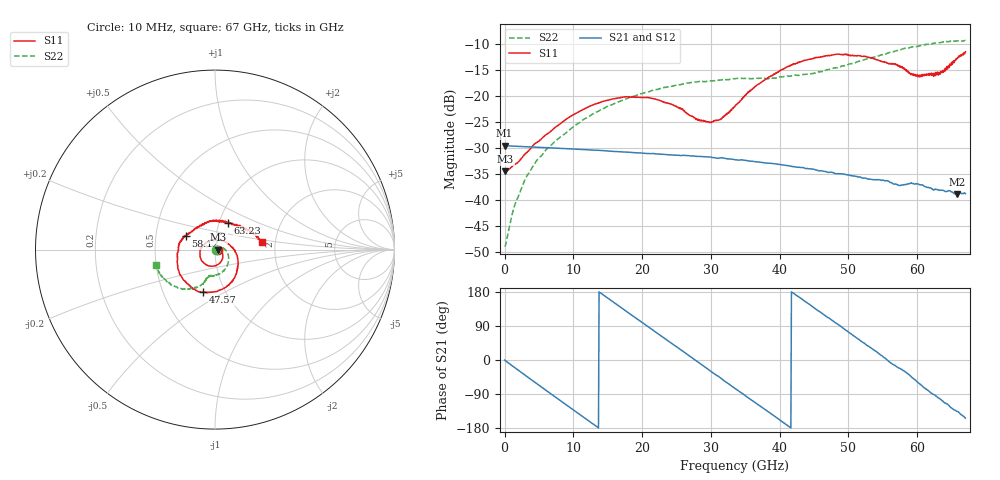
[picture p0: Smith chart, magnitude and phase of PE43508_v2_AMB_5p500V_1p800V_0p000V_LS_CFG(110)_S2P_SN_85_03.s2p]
!Keysight Technologies,N5227A,US51270237,A.10.43.00
!Date: Wednesday, August 22, 2018 17:18:10
!Correction: S11(Full 2 Port(1,3))
!S31(Full 2 Port(1,3))
!S13(Full 2 Port(1,3))
!S33(Full 2 Port(1,3))
!S2P File: Measurements: S11, S31, S13, S33:
# Hz S  dB  R 50
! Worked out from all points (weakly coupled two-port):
!   801 points, 10 MHz to 67 GHz, reference 50 ohm
!   highest |S21| = -29.57 dB at 10 MHz (marker M1); lowest = -38.9 dB at 65.83 GHz (marker M2)
!   lowest |S11| = -34.5 dB at 93.74 MHz (marker M3), VSWR 1.04, Z = 51.9 + j0.00866 ohm
!   |S11| at or under -10 dB: start of sweep to end of sweep
!   |S22| runs from -48.9 to -9.3 dB; largest |S21 - S12| = 0.0002
!   S11 on the Smith chart (normalised r, x): 10 MHz: 1.04, -0.00; 47.57 GHz: 0.79, -0.40; 58.12 GHz: 0.71, +0.11; 63.23 GHz: 1.10, +0.34; 67 GHz: 1.70, +0.15
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1e7  -34.43 -1.1  -29.57 -0.2  -29.58 -0.2  -48.82 -2.1
9.37375e7  -34.50 0.3  -29.59 -1.4  -29.60 -1.4  -48.90 7.8
1.68475e9  -33.03 3.3  -29.70 -22.8  -29.70 -22.9  -40.24 46.7
3.02455e9  -31.17 -0.3  -29.78 -40.6  -29.78 -40.6  -35.96 43.8
4.36435e9  -29.25 -7.2  -29.86 -58.2  -29.86 -58.2  -33.03 37.6
7.295162e9  -26.14 -28.8  -30.05 -96.6  -30.05 -96.5  -28.81 23.4
1.123082e10  -22.73 -61.1  -30.31 -147.7  -30.32 -147.7  -24.82 -1.0
1.74274e10  -20.22 -111.6  -30.78 132.2  -30.78 132.2  -20.68 -34.1
2.236791e10  -20.78 -154.8  -31.20 68.5  -31.19 68.5  -18.70 -57.0
2.973681e10  -25.07 96.9  -31.76 -26.3  -31.76 -26.3  -17.10 -82.8
3.132782e10  -24.56 63.7  -31.93 -46.3  -31.94 -46.3  -16.94 -87.6
3.3505e10  -22.04 24.3  -32.27 -75.1  -32.28 -75.2  -16.69 -93.3
3.836178e10  -16.49 -30.9  -32.96 -136.8  -32.97 -136.8  -16.68 -100.8
4.472582e10  -12.87 -83.7  -34.07 141.3  -34.06 141.3  -15.73 -105.3
4.75729e10  -12.14 -105.6  -34.70 105.1  -34.69 105.0  -14.75 -107.7
5.234594e10  -12.38 -144.0  -35.80 43.6  -35.79 43.4  -13.03 -113.3
5.586291e10  -13.87 -179.4  -36.46 -3.9  -36.44 -4.3  -11.69 -122.6
5.812382e10  -14.94 155.2  -37.08 -29.5  -37.09 -30.0  -10.90 -129.4
6.004979e10  -15.96 122.3  -36.93 -58.1  -36.92 -58.5  -10.50 -136.3
6.323181e10  -15.53 64.4  -38.12 -101.7  -38.11 -102.3  -9.79 -149.2
6.582768e10  -12.72 24.1  -38.94 -135.8  -39.01 -136.0  -9.45 -159.1
6.7e10  -11.50 8.8  -38.82 -153.3  -38.90 -153.3  -9.36 -165.4
